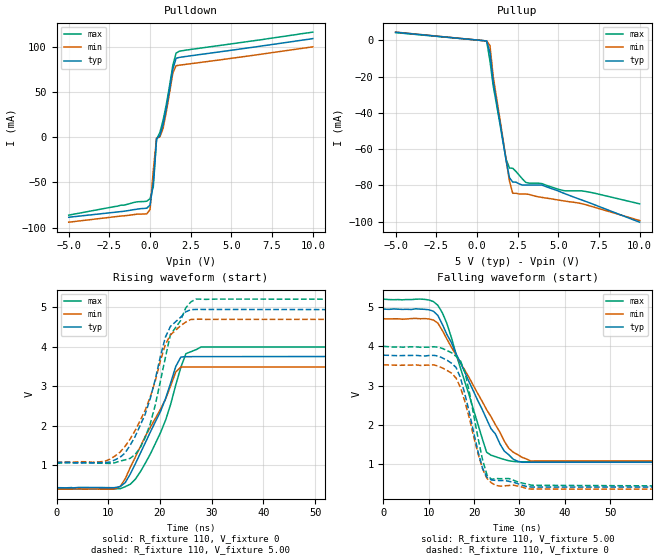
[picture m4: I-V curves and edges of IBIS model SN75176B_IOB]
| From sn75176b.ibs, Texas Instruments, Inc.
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|   Model SN75176B_IOB
[Model]   SN75176B_IOB
Model_type  I/O
Polarity   Inverting
Enable   Active-High
Vinl = 2.2
Vinh = 2.8
| variable   typ   min   max
C_comp   14.112pf   12.360pf   14.223pf
[Temperature Range]   40   0   85
| Ambient temperature   25   0   70
[Voltage Range]   5.00   4.75   5.25
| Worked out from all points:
|   slope of the pulldown table from 0 to 0.75 V, typ, clamps not added: 8.73 ohm
|   slope of the pullup table from 0 to 0.75 V, typ, clamps not added: 140 ohm
|   rising waveform, R_fixture 110, V_fixture 0: 20-80 % time 6.63ns typ, 7.14ns min, 6.14ns max; typ from 0.43 V to 3.75 V
|   falling waveform, R_fixture 110, V_fixture 5.00: 20-80 % time 9.62ns typ, 10.7ns min, 6.6ns max; typ from 4.95 V to 1.05 V
|   rising waveform, R_fixture 110, V_fixture 5.00: 20-80 % time 5.31ns typ, 5.99ns min, 4.74ns max; typ from 1.07 V to 4.95 V
|   falling waveform, R_fixture 110, V_fixture 0: 20-80 % time 4.19ns typ, 4.42ns min, 3.72ns max; typ from 3.78 V to 0.423 V
[Pulldown]
|   Voltage   I(typ)   I(min)   I(max)
-5V       -88.68mA   -94.13mA   -86.33mA
-200mV    -78.65mA   -84.9mA    -70.92mA
0V        -75.16mA   -80.07mA   -68.17mA
200mV     -50.16mA   -36.86mA   -54.7mA
400mV     -1.786mA   -960.3uA   -2.31mA
600mV     1.463mA    -130.5uA   4.87mA
800mV     13.8mA     9.488mA    18.53mA
1V        31.84mA    27.92mA    36.08mA
1.4V      75.01mA    70.88mA    79.19mA
1.6V      87.06mA    78.84mA    92.77mA
2V        88.55mA    79.88mA    95.48mA
10V       108.8mA    99.68mA    116mA
[Pullup]
|   Voltage   I(typ)   I(min)   I(max)
-5V       4.497mA    4.59mA     4.307mA
600mV     -323.8uA   -325uA     -422.5uA
800mV     -6.738mA   -2.755mA   -11.39mA
1V        -22.79mA   -19.92mA   -25.11mA
1.8V      -66.71mA   -66.15mA   -65.79mA
2V        -75.74mA   -77.68mA   -70.41mA
2.2V      -78.17mA   -84.34mA   -70.57mA
3V        -79.82mA   -84.74mA   -78.32mA
4V        -79.82mA   -86.64mA   -79.04mA
5.4V      -84.55mA   -88.64mA   -82.98mA
6.4V      -87.91mA   -90mA      -82.98mA
10V       -100.3mA   -99.39mA   -90.17mA
[Ramp]
| variable   typ   min   max
dV/dt_r  2.04E+00/6.70E-09  2.07E+00/7.70E-09  2.20E+00/6.20E-09
dV/dt_f  2.06E+00/4.30E-09  2.04E+00/4.80E-09  2.05E+00/3.61E-09
R_load = 110
[Rising Waveform]
R_fixture = 110
V_fixture = 0
V_fixture_min = 0
V_fixture_max = 0
C_fixture = 0pf
L_fixture = 0nH
|   Time   V(typ)   V(min)   V(max)
0s        430.5mV    393.5mV    400.5mV
11.15ns   429.8mV    395.8mV    400.4mV
12.32ns   458.1mV    463.1mV    404.6mV
14.27ns   778.8mV    947.7mV    517.6mV
20.13ns   2.369V     2.426V     1.831V
23.06ns   3.503V     3.362V     3.034V
24.04ns   3.739V     3.487V     3.48V
25.02ns   3.748V     3.487V     3.824V
27.97ns   3.75V      3.487V     3.996V
75.2ns    3.75V      3.487V     3.996V
[Falling Waveform]
R_fixture = 110
V_fixture = 5.00
V_fixture_min = 4.75
V_fixture_max = 5.25
C_fixture = 0pf
L_fixture = 0nH
|   Time   V(typ)   V(min)   V(max)
0s        4.951V     4.703V     5.203V
10.06ns   4.933V     4.701V     5.182V
12.02ns   4.788V     4.593V     5.046V
13.97ns   4.312V     4.196V     4.593V
22.76ns   2.15V      2.391V     1.308V
23.73ns   1.907V     2.213V     1.235V
27.64ns   1.245V     1.409V     1.093V
29.59ns   1.081V     1.248V     1.066V
32.52ns   1.054V     1.086V     1.066V
75.2ns    1.054V     1.089V     1.066V
[Rising Waveform]
R_fixture = 110
V_fixture = 5.00
V_fixture_min = 4.75
V_fixture_max = 5.25
C_fixture = 0pf
L_fixture = 0nH
|   Time   V(typ)   V(min)   V(max)
0s        1.066V     1.074V     1.049V
10.3ns    1.077V     1.149V     1.044V
13.23ns   1.305V     1.473V     1.133V
15.18ns   1.722V     1.872V     1.266V
18.11ns   2.685V     2.724V     2.042V
21.04ns   4.239V     4.057V     3.723V
22.02ns   4.515V     4.299V     4.304V
24.97ns   4.883V     4.622V     4.981V
26.92ns   4.945V     4.696V     5.208V
75.2ns    4.947V     4.689V     5.2V
[Falling Waveform]
R_fixture = 110
V_fixture = 0
V_fixture_min = 0
V_fixture_max = 0
C_fixture = 0pf
L_fixture = 0nH
|   Time   V(typ)   V(min)   V(max)
0s        3.778V     3.532V     4.003V
12.11ns   3.756V     3.496V     3.981V
16.02ns   3.466V     3.195V     3.75V
16.99ns   3.206V     2.957V     3.635V
18.95ns   2.32V      2.17V      2.84V
21.88ns   895.1mV    884.4mV    1.108V
22.85ns   667.7mV    640mV      728.5mV
23.83ns   602.9mV    528.7mV    621.2mV
32.62ns   423.5mV    372.7mV    471mV
75.2ns    423.3mV    370.9mV    445.7mV
